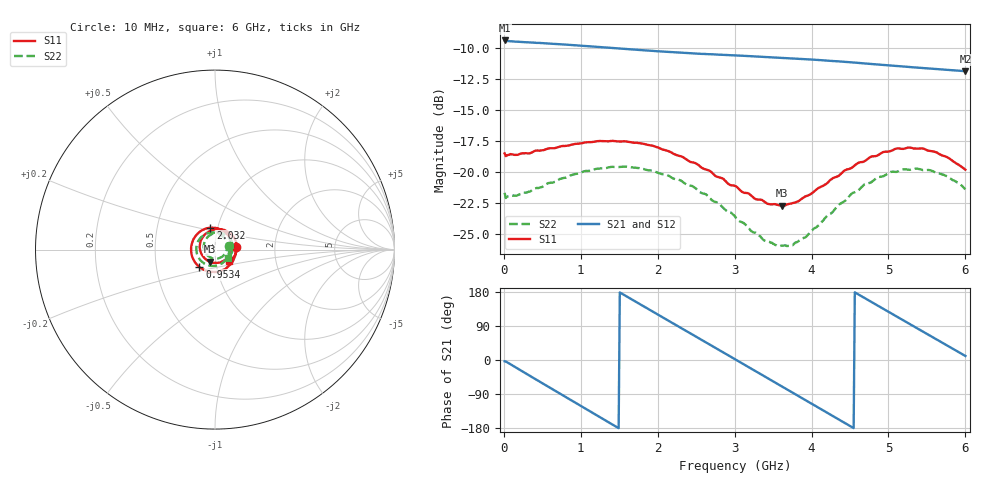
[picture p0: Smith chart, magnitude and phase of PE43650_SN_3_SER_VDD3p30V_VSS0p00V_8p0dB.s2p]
!Keysight Technologies,N5245B,MY57181451,A.13.50.07
!Date: Tuesday, May 07, 2019 08:00:00
!Correction: S11(Full 2 Port(1,2))
!S21(Full 2 Port(1,2))
!S12(Full 2 Port(1,2))
!S22(Full 2 Port(1,2))
!S2P File: Measurements: S11, S21, S12, S22:
# Hz S  dB  R 50
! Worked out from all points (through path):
!   401 points, 10 MHz to 6 GHz, reference 50 ohm
!   highest |S21| = -9.36 dB at 10 MHz (marker M1); lowest = -11.8 dB at 6 GHz (marker M2)
!   group delay of S21, straight-line fit = 328 ps
!   lowest |S11| = -22.7 dB at 3.619 GHz (marker M3), VSWR 1.16, Z = 46.8 - j6.29 ohm
!   |S11| at or under -10 dB: start of sweep to end of sweep
!   |S22| runs from -26.0 to -19.6 dB; largest |S21 - S12| = 0.0033
!   S11 on the Smith chart (normalised r, x): 10 MHz: 1.27, +0.04; 953.4 MHz: 0.83, -0.16; 2.032 GHz: 0.92, +0.23; 6 GHz: 1.16, -0.15
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1e7  -18.49 6.8  -9.36 -3.4  -9.44 -3.3  -21.68 12.9
2.496e8  -18.48 -36.9  -9.49 -31.0  -9.54 -31.0  -21.66 -37.2
5.1915e8  -18.23 -75.0  -9.58 -63.6  -9.62 -63.6  -21.13 -76.5
7.43775e8  -17.92 -104.9  -9.67 -90.7  -9.72 -90.7  -20.55 -105.8
9.53425e8  -17.71 -131.8  -9.76 -115.8  -9.81 -115.8  -20.14 -132.3
1.013325e9  -17.67 -139.5  -9.79 -123.0  -9.84 -123.0  -20.02 -139.6
1.2679e9  -17.50 -170.1  -9.90 -153.3  -9.96 -153.3  -19.71 -168.8
1.5075e9  -17.54 161.4  -10.01 178.2  -10.07 178.3  -19.59 164.4
1.7471e9  -17.65 134.1  -10.12 149.9  -10.18 149.9  -19.68 138.8
2.01665e9  -18.05 103.7  -10.24 118.2  -10.29 118.2  -20.10 110.4
2.031625e9  -18.09 102.0  -10.24 116.4  -10.30 116.4  -20.13 108.7
2.4659e9  -19.24 51.3  -10.41 65.4  -10.46 65.4  -21.20 62.1
2.750425e9  -20.33 16.8  -10.49 32.0  -10.55 32.1  -22.42 29.2
3.005e9  -21.13 -17.6  -10.56 2.1  -10.62 2.1  -23.60 -2.4
3.289525e9  -22.22 -59.9  -10.65 -31.5  -10.70 -31.4  -24.98 -44.8
3.618975e9  -22.74 -113.5  -10.76 -70.3  -10.81 -70.2  -25.95 -101.1
4.008325e9  -21.70 -176.2  -10.90 -116.2  -10.95 -116.2  -24.72 -168.7
4.5025e9  -19.72 116.7  -11.12 -174.5  -11.18 -174.3  -21.88 122.2
4.7421e9  -18.89 87.8  -11.24 157.4  -11.30 157.5  -20.90 95.0
5.01165e9  -18.33 58.3  -11.38 125.9  -11.43 126.0  -20.05 65.2
5.4609e9  -18.12 12.0  -11.59 73.4  -11.64 73.6  -19.85 19.7
6e9  -19.81 -39.6  -11.84 10.6  -11.89 10.7  -21.40 -31.6
